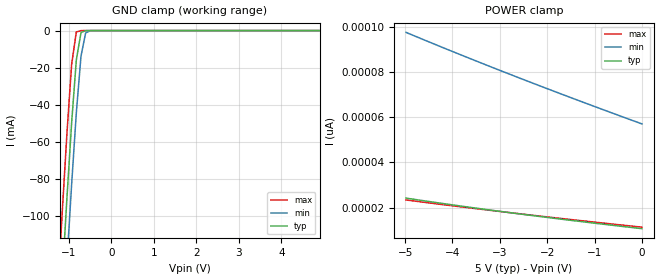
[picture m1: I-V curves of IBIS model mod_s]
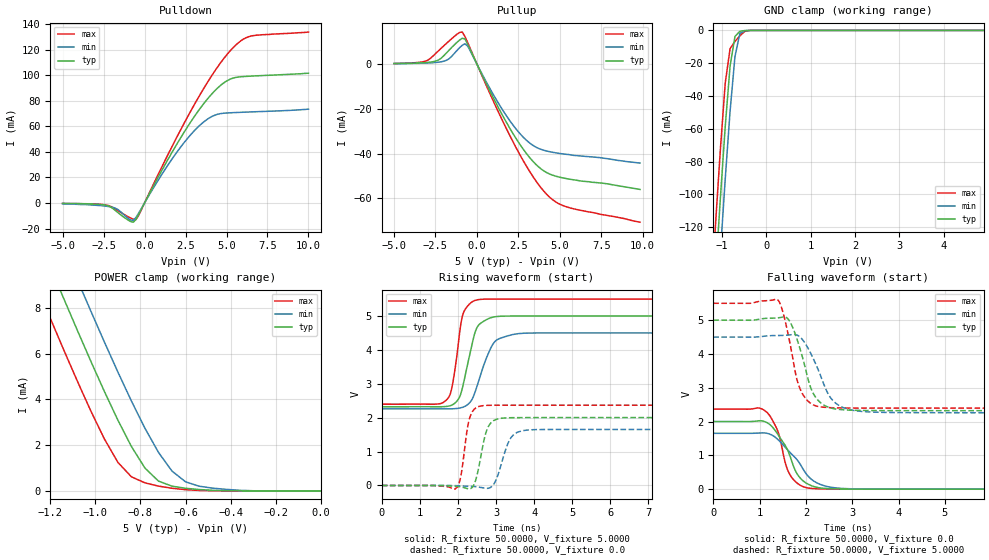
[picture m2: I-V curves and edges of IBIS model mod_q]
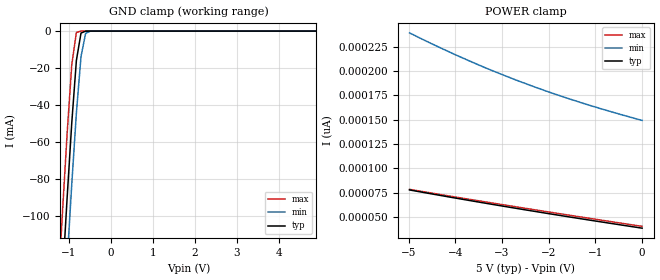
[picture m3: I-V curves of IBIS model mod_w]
| IBIS (I/O, Buffer, Information, Specification) Model, officially
| electronic behavioral standard for Buffer structures of digital pins.
[IBIS ver]  4.0
[File name] m95xxx_c6_tssop8.ibs
[File Rev]  1.0
[Date]   22 July 2016
[Source]   CAD & Design Services (Catania) - STMicroelectronics
[Notes]
   (Note1)  This IBIS model includes the SO8 ceramic package parasitic data
   (Note2)  This IBIS model considers: VCC= 5.00(TYP), 4.50(MIN), 5.50(MAX)
   (Note3)  This IBIS model has some Notes about the non-monotonicity
   of the I-V curves, but they are not indicative of problems
   inside the model;
[Copyright] (c) 2016 STMicroelectronics
|   Component M95XXX
[Component] M95XXX
[Manufacturer] STMicroelectronics
[Package]
| variable   typ   min   max
R_pkg   0.0   0.0   0.0
L_pkg   0.0H   0.0H   0.0H
C_pkg   0.0F   0.0F   0.0F
[Pin]  signal_name   model_name   R_pin   L_pin   C_pin
1   SN   mod_s   NA   NA   NA
2   Q   mod_q   NA   NA   NA
3   WN   mod_w   NA   NA   NA
4   GND   GND   NA   NA   NA
5   D   mod_s   NA   NA   NA
6   C   mod_s   NA   NA   NA
7   HOLDN   mod_h   NA   NA   NA
8   VCCIO   POWER   NA   NA   NA
[Package Model]  182696_TSSOP8
[Define Package Model]  182696_TSSOP8
[Manufacturer]  STMicroelectronics
[OEM]  STMicroelectronics
[Description]  8 pin TSSOP package
[Number Of Pins]  8
[Pin Numbers]
|Pin Num   Terminal Name
1   | net1
2   | net2
3   | net3
4   | net4_GND
5   | net5
6   | net6
7   | net7
8   | net8_VDD
[Model Data]
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[End Model Data]
[End Package Model]
| Models and submodels in the file (4): mod_s (Input), mod_q (I/O), mod_w (Input), mod_h (Input)
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|   Model mod_s
[Model]   mod_s
Model_type Input
Vinl   =   1.250V
Vinh   =   3.750V
C_comp   2.119pF   2.024pF   2.324pF
[Temperature Range]  25.0000   85.0000   -40.0000
[Voltage Range]   5.0000V   4.5000V   5.5000V
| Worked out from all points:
|   GND clamp passes 1 mA (typ) near -0.70 V on its own axis
[GND_clamp]
|Voltage   I(typ)   I(min)   I(max)
-5V       -1.764A    -1.796A    -1.733A
-1.26V    -176.7mA   -211.6mA   -141.2mA
-1.15V    -132.7mA   -167.5mA   -97.27mA
-1.04V    -89.88mA   -124.3mA   -55.14mA
-930mV    -49.58mA   -82.71mA   -18.16mA
-820mV    -15.87mA   -44.29mA   -757uA
-710mV    -1.068mA   -13.78mA   -5.45uA
-600mV    -23.1uA    -1.246mA   -36.27nA
-490mV    -459.2nA   -51.76uA   -242.2pA
4.9V      10.56pA    60.08pA    10.13pA
[POWER_clamp]
|Voltage   I(typ)   I(min)   I(max)
-4.98V    24.27pA    97.43pA    23.46pA
-3.84V    20.82pA    87.65pA    20.47pA
-2.58V    17.29pA    77.24pA    17.36pA
-1.32V    14.01pA    67.21pA    14.4pA
0V        10.79pA    57.03pA    11.44pA
|   Model mod_q
[Model]   mod_q
Model_type I/O
Polarity   Non-Inverting
Enable   Active-Low
Vinl   =   1.250V
Vinh   =   3.750V
Vmeas  =   2.500V
Cref   =   30pF
C_comp   2.668pF   2.548pF   2.925pF
[Temperature Range]  25.0000   85.0000   -40.0000
[Voltage Range]   5.0000V   4.5000V   5.5000V
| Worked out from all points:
|   slope of the pulldown table from 0 to 0.75 V, typ, clamps not added: 41 ohm
|   slope of the pullup table from 0 to 0.75 V, typ, clamps not added: 64.9 ohm
|   GND clamp passes 1 mA (typ) near -0.62 V on its own axis
|   POWER clamp passes 1 mA (typ) near -0.78 V on its own axis
|   rising waveform, R_fixture 50.0000, V_fixture 5.0000: 20-80 % time 322ps typ, 427ps min, 231ps max; typ from 2.32 V to 5 V
|   rising waveform, R_fixture 50.0000, V_fixture 0.0: 20-80 % time 227ps typ, 291ps min, 180ps max; typ from 0 V to 2 V
|   falling waveform, R_fixture 50.0000, V_fixture 0.0: 20-80 % time 432ps typ, 587ps min, 304ps max; typ from 2 V to 0 V
|   falling waveform, R_fixture 50.0000, V_fixture 5.0000: 20-80 % time 348ps typ, 439ps min, 290ps max; typ from 5 V to 2.32 V
[Pulldown]
|Voltage   I(typ)   I(min)   I(max)
-5V       -300uA     -700uA     -300uA
-2.28V    -2.04mA    -2.63mA    -1.78mA
-1.64V    -7.36mA    -5.01mA    -5.87mA
-840mV    -14.57mA   -13.33mA   -11.84mA
-520mV    -12.8mA    -11.32mA   -12.96mA
1.4V      33.44mA    29.18mA    37.15mA
2.84V     63.92mA    53.82mA    72.48mA
4.12V     85.6mA     67.79mA    100.1mA
5.24V     97.05mA    70.62mA    119.4mA
5.88V     98.83mA    70.99mA    127mA
6.52V     99.34mA    71.31mA    130.8mA
10V       101.6mA    73.46mA    133.8mA
[Pullup]
|Voltage   I(typ)   I(min)   I(max)
-5V       220uA      170uA      270uA
-3.12V    642uA      426uA      1.259mA
-2.48V    1.34mA     705uA      4.783mA
-1.68V    6.188mA    2.366mA    10.3mA
-880mV    11.53mA    8.413mA    14.28mA
-560mV    8.919mA    8.049mA    9.648mA
1.04V     -15.82mA   -14.26mA   -17.33mA
2.32V     -32.77mA   -28.63mA   -36.74mA
3.28V     -42.61mA   -35.8mA    -49.1mA
4.24V     -48.6mA    -38.91mA   -58.41mA
5.52V     -51.33mA   -40.4mA    -64.04mA
9.84V     -56mA      -44.22mA   -70.64mA
[GND_clamp]
|Voltage   I(typ)   I(min)   I(max)
-5V       -1.918A    -1.948A    -1.89A
-1.15V    -149.1mA   -182.6mA   -118.8mA
-1.04V    -102.6mA   -135.8mA   -72.9mA
-930mV    -58.74mA   -90.78mA   -32.17mA
-820mV    -21.58mA   -49.1mA    -11.08mA
-710mV    -3.653mA   -15.88mA   -6.723mA
-600mV    -555.3uA   -1.844mA   -3.311mA
-490mV    -79.08uA   -228.4uA   -612.8uA
-380mV    -6.392uA   -39.85uA   -6.411uA
4.9V      216.5pA    54.61uA    174.3pA
[POWER_clamp]
|Voltage   I(typ)   I(min)   I(max)
-4.98V    102.8mA    104.9mA    100.8mA
-1.26V    11.22mA    13.44mA    8.958mA
-1.2V     9.805mA    12.03mA    7.55mA
-1.14V    8.405mA    10.62mA    6.161mA
-1.08V    7.024mA    9.234mA    4.803mA
-1.02V    5.669mA    7.861mA    3.493mA
-900mV    3.093mA    5.197mA    1.249mA
-780mV    999.4uA    2.74mA     353uA
-660mV    208.6uA    867.2uA    116.3uA
-600mV    115.4uA    399.5uA    55.12uA
-480mV    28.08uA    121.3uA    6.586uA
0V        230.6pA    776.4pA    241.5pA
[Ramp]
| variable   typ   min   max
dV/dt_r  1.2015/0.2702n   0.9918/0.3464n   1.4213/0.2190n
dV/dt_f  1.6073/0.3921n   1.3425/0.4932n   1.8614/0.3216n
R_load = 50.0000
[Rising Waveform]
R_fixture= 50.0000
V_fixture= 5.0000
V_fixture_min= 4.5000
V_fixture_max= 5.5000
|time   V(typ)   V(min)   V(max)
0s        2.323V     2.262V     2.398V
1.72ns    2.335V     2.261V     2.55V
1.86ns    2.384V     2.263V     3.001V
2.02ns    2.563V     2.28V      4.284V
2.12ns    2.891V     2.306V     5.01V
2.34ns    4.013V     2.488V     5.392V
2.48ns    4.613V     2.857V     5.47V
2.92ns    4.966V     4.172V     5.5V
3.46ns    5V         4.459V     5.5V
10ns      5V         4.5V       5.5V
[Rising Waveform]
R_fixture= 50.0000
V_fixture= 0.0
V_fixture_min= 0.0
V_fixture_max= 0.0
|time   V(typ)   V(min)   V(max)
0s        7.837nV    63.42nV    7.911nV
1.92ns    -25.1mV    -4.851mV   -109.1mV
2.07ns    -42.26mV   -11.34mV   244.3mV
2.31ns    -99.76mV   -25.26mV   2.001V
2.45ns    104.7mV    -35.05mV   2.272V
2.59ns    794.4mV    -55.99mV   2.342V
2.87ns    1.853V     -46.38mV   2.366V
3.35ns    1.998V     1.331V     2.368V
3.69ns    2.002V     1.616V     2.368V
10ns      2.002V     1.653V     2.368V
[Falling Waveform]
R_fixture= 50.0000
V_fixture= 0.0
V_fixture_min= 0.0
V_fixture_max= 0.0
|time   V(typ)   V(min)   V(max)
0s        2.002V     1.653V     2.368V
1.13ns    1.989V     1.661V     2.307V
1.39ns    1.632V     1.476V     1.73V
1.55ns    1.302V     1.247V     805.8mV
1.65ns    1.009V     1.097V     442.1mV
1.81ns    455.6mV    869.4mV    180.8mV
2.05ns    146.5mV    382.6mV    34.76mV
2.34ns    31.65mV    126.8mV    7.444mV
2.89ns    3.705mV    14.87mV    573.2uV
10ns      8.216nV    -16.42nV   -37.57nV
[Falling Waveform]
R_fixture= 50.0000
V_fixture= 5.0000
V_fixture_min= 4.5000
V_fixture_max= 5.5000
|time   V(typ)   V(min)   V(max)
0s        5V         4.5V       5.5V
1.4ns     5.071V     4.546V     5.595V
1.5ns     5.093V     4.55V      5.258V
1.62ns    5.028V     4.56V      4.562V
1.86ns    4.214V     4.517V     3.016V
2.1ns     3.019V     4.031V     2.543V
2.26ns    2.634V     3.553V     2.449V
2.6ns     2.382V     2.598V     2.408V
3.16ns    2.33V      2.306V     2.399V
10ns      2.323V     2.262V     2.398V
|   Model mod_w
[Model]   mod_w
Model_type Input
Vinl   =   1.250V
Vinh   =   3.750V
C_comp   2.119pF   2.024pF   2.324pF
[Temperature Range]  25.0000   85.0000   -40.0000
[Voltage Range]   5.0000V   4.5000V   5.5000V
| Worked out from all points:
|   GND clamp passes 1 mA (typ) near -0.70 V on its own axis
[GND_clamp]
|Voltage   I(typ)   I(min)   I(max)
-5V       -1.764A    -1.796A    -1.733A
-1.26V    -176.7mA   -211.6mA   -141.2mA
-1.15V    -132.7mA   -167.5mA   -97.27mA
-1.04V    -89.88mA   -124.3mA   -55.14mA
-930mV    -49.58mA   -82.71mA   -18.16mA
-820mV    -15.87mA   -44.29mA   -757uA
-710mV    -1.068mA   -13.78mA   -5.45uA
-600mV    -23.1uA    -1.246mA   -36.27nA
-490mV    -459.2nA   -51.76uA   -242.2pA
4.9V      10.56pA    60.08pA    10.13pA
[POWER_clamp]
|Voltage   I(typ)   I(min)   I(max)
-4.98V    77.79pA    239.4pA    78.35pA
-4.5V     73.66pA    228.1pA    74.49pA
-3.9V     68.61pA    214.8pA    69.73pA
-3.18V    62.72pA    200pA      64.11pA
-2.58V    57.92pA    188.7pA    59.5pA
-1.86V    52.32pA    176.3pA    54.05pA
-1.32V    48.2pA     167.8pA    50.01pA
-660mV    43.28pA    158.2pA    45.13pA
0V        38.45pA    149.3pA    40.3pA
